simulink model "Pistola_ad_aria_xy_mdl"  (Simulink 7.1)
settings: Solver=ode45  StartTime=0.0  StopTime=10.0  RelTol=1e-6
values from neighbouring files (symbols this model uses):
  A0 = 2*cm^2    (= 0.0002)    [Pistola_ad_aria_xy.m]
  AngS = 10*gradi    (= 0.174532925199)    [Pistola_ad_aria_xy.m]
  Ap = 0.3*cm^2    (= 3e-05)    [Pistola_ad_aria_xy.m]
  b0 = 0.8*N/(10*cm/sec)    (= 8)    [Pistola_ad_aria_xy.m]
  Bp = eye(2)*bp    [Pistola_ad_aria_xy.m]
  bt = bm+b1*(r0/r1)^2+b3*(r0*r2/(r1*r3))^2+b5*(r0*r2*r4/(r1*r3*r5))^2    (= 0.0109583333333)    [Pistola_ad_aria_xy.m]
  g = 9.81*m/sec^2    (= 9.81)    [Pistola_ad_aria_xy.m]
  Imax = 10000*Amp    (= 10000)    [Pistola_ad_aria_xy.m]
  Jt = Jm+J1*(r0/r1)^2+J3*(r0*r2/(r1*r3))^2+J5*(r0*r2*r4/(r1*r3*r5))^2    (= 3.6984375e-05)    [Pistola_ad_aria_xy.m]
  K0 = 1*800*N/(5*cm)    (= 16000)    [Pistola_ad_aria_xy.m]
  K7 = 100*N/(1*mm)    (= 100000)    [Pistola_ad_aria_xy.m]
  Ke = 0.5*N*m/Amp    (= 0.5)    [Pistola_ad_aria_xy.m]
  La = 0.05*Henry    (= 0.05)    [Pistola_ad_aria_xy.m]
  m0 = 50*gr    (= 0.05)    [Pistola_ad_aria_xy.m]
  mp = 10*gr    (= 0.01)    [Pistola_ad_aria_xy.m]
  Mp = eye(2)*mp    [Pistola_ad_aria_xy.m]
  P0 = 1*bar    (= 100000)    [Pistola_ad_aria_xy.m]
  r6 = 3.5*r0    (= 0.035)    [Pistola_ad_aria_xy.m]
  Ra = 2*Ohm    (= 2)    [Pistola_ad_aria_xy.m]
  rt = r0*r2*r4/(r1*r3*r5)    (= 0.0416666666667)    [Pistola_ad_aria_xy.m]
  Tau_r = 0*N*m    (= 0)    [Pistola_ad_aria_xy.m]
  Tc = Tfin/8000    (= 0.000625)    [Pistola_ad_aria_xy.m]
  Th3_0 = 0    [Pistola_ad_aria_xy.m]
  V0 = pi*r6*A0    (= 2.19911485751e-05)    [Pistola_ad_aria_xy.m]
  Va = 30*V    (= 30)    [Pistola_ad_aria_xy.m]
  XP_0 = [0; 1.5]*m    [Pistola_ad_aria_xy.m]

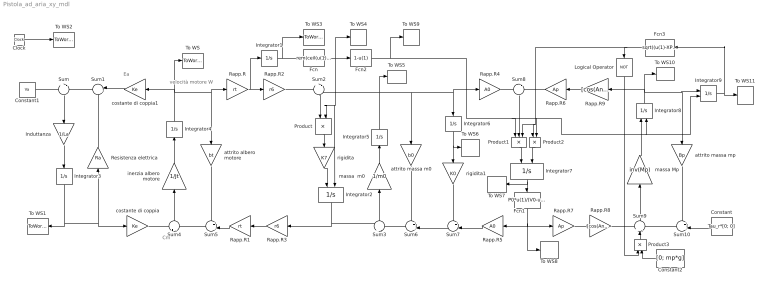
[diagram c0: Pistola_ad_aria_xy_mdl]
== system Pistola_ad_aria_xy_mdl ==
  note: Ea
  note: velocità motore W
  note: Cm
  Clock : Clock
  Constant : Constant  Orientation=left  Value=Tau_r*[0; 0]  OutDataType=sfix(16)  OutScaling=2^0
  Constant1 : Constant  Value=Va  OutDataType=sfix(16)  OutScaling=2^0
  Constant2 : Constant  Orientation=left  Value=[0; mp*g]  OutDataType=sfix(16)  OutScaling=2^0
  Fcn : Fcn  Expr=rem(ceil(u(1)/pi),2)
  Fcn1 : Fcn  Orientation=down  Expr=P0*u(1)/(V0-u(1))
  Fcn2 : Fcn  Expr=1-u(1)
  Fcn3 : Fcn  Orientation=left  Expr=sqrt((u(1)-XP_0(1))^2+(u(2)-XP_0(2))^2)<Lung_Canna
  Induttanza : Gain  Orientation=down  Gain=1/La  ParameterDataType=sfix(16)  ParameterScaling=2^0  OutDataType=sfix(16)  OutScaling=2^0
  Integrator1 : Integrator  InitialCondition=Th3_0
  Integrator2 : Integrator  Orientation=down  ExternalReset=falling
  Integrator3 : Integrator  Orientation=down  UpperSaturationLimit=Imax  LowerSaturationLimit=-Imax
  Integrator4 : Integrator  Orientation=up
  Integrator5 : Integrator  Orientation=up
  Integrator6 : Integrator  Orientation=down
  Integrator7 : Integrator  Orientation=down  ExternalReset=either
  Integrator8 : Integrator  Orientation=up  ExternalReset=rising
  Integrator9 : Integrator  ExternalReset=rising  InitialCondition=XP_0
  Logical Operator : Logic  Orientation=down  Operator=NOT  AllPortsSameDT=off  OutDataTypeMode=boolean  OutDataTypeStr=boolean
  Product : Product  Orientation=down  OutDataType=sfix(16)  OutScaling=2^0
  Product1 : Product  Orientation=down  Inputs=3  OutDataType=sfix(16)  OutScaling=2^0
  Product2 : Product  Orientation=down  OutDataType=sfix(16)  OutScaling=2^0
  Product3 : Product  Orientation=up  OutDataType=sfix(16)  OutScaling=2^0
  Rapp.R : Gain  Gain=rt  ParameterDataType=sfix(16)  ParameterScaling=2^0  OutDataType=sfix(16)  OutScaling=2^0
  Rapp.R1 : Gain  Orientation=left  Gain=rt  ParameterDataType=sfix(16)  ParameterScaling=2^0  OutDataType=sfix(16)  OutScaling=2^0
  Rapp.R2 : Gain  Gain=r6  ParameterDataType=sfix(16)  ParameterScaling=2^0  OutDataType=sfix(16)  OutScaling=2^0
  Rapp.R3 : Gain  Orientation=left  Gain=r6  ParameterDataType=sfix(16)  ParameterScaling=2^0  OutDataType=sfix(16)  OutScaling=2^0
  Rapp.R4 : Gain  Gain=A0  ParameterDataType=sfix(16)  ParameterScaling=2^0  OutDataType=sfix(16)  OutScaling=2^0
  Rapp.R5 : Gain  Orientation=left  Gain=A0  ParameterDataType=sfix(16)  ParameterScaling=2^0  OutDataType=sfix(16)  OutScaling=2^0
  Rapp.R6 : Gain  Orientation=left  Gain=Ap  ParameterDataType=sfix(16)  ParameterScaling=2^0  OutDataType=sfix(16)  OutScaling=2^0
  Rapp.R7 : Gain  Gain=Ap  ParameterDataType=sfix(16)  ParameterScaling=2^0  OutDataType=sfix(16)  OutScaling=2^0
  Rapp.R8 : Gain  Gain=[cos(AngS); sin(AngS)]  Multiplication=Matrix(K*u)  ParameterDataType=sfix(16)  ParameterScaling=2^0  OutDataType=sfix(16)  OutScaling=2^0
  Rapp.R9 : Gain  Orientation=left  Gain="[cos(AngS)  sin(AngS)]"  Multiplication=Matrix(K*u)  ParameterDataType=sfix(16)  ParameterScaling=2^0  OutDataType=sfix(16)  OutScaling=2^0
  Resistenza elettrica : Gain  Orientation=up  Gain=Ra  ParameterDataType=sfix(16)  ParameterScaling=2^0  OutDataType=sfix(16)  OutScaling=2^0
  Sum : Sum  Orientation=down  Inputs=+|-  OutDataType=sfix(16)  OutScaling=2^0
  Sum1 : Sum  Orientation=left  Inputs=|++  OutDataType=sfix(16)  OutScaling=2^0
  Sum10 : Sum  Orientation=left  Inputs=++|  OutDataType=sfix(16)  OutScaling=2^0
  Sum2 : Sum  Orientation=down  Inputs=+|-  OutDataType=sfix(16)  OutScaling=2^0
  Sum3 : Sum  Orientation=up  Inputs=+|-  OutDataType=sfix(16)  OutScaling=2^0
  Sum4 : Sum  Orientation=up  Inputs=+|-  OutDataType=sfix(16)  OutScaling=2^0
  Sum5 : Sum  Orientation=left  Inputs=++|  OutDataType=sfix(16)  OutScaling=2^0
  Sum6 : Sum  Orientation=left  Inputs=++|  OutDataType=sfix(16)  OutScaling=2^0
  Sum7 : Sum  Orientation=left  Inputs=+-|  OutDataType=sfix(16)  OutScaling=2^0
  Sum8 : Sum  Orientation=down  Inputs=-|-  OutDataType=sfix(16)  OutScaling=2^0
  Sum9 : Sum  Orientation=up  Inputs=+--  OutDataType=sfix(16)  OutScaling=2^0
  To WS : ToWorkspace  VariableName=Wm  SampleTime=Tc  SaveFormat=Array
  To WS1 : ToWorkspace  VariableName=Ia  SampleTime=Tc  SaveFormat=Array
  To WS10 : ToWorkspace  VariableName=XPdot  SampleTime=Tc  SaveFormat=Array
  To WS11 : ToWorkspace  VariableName=XP  SampleTime=Tc  SaveFormat=Array
  To WS2 : ToWorkspace  VariableName=t  SampleTime=Tc  SaveFormat=Array
  To WS3 : ToWorkspace  VariableName=Th3  SampleTime=Tc  SaveFormat=Array
  To WS4 : ToWorkspace  VariableName=Car  SampleTime=Tc  SaveFormat=Array
  To WS5 : ToWorkspace  VariableName=X0dot  SampleTime=Tc  SaveFormat=Array
  To WS6 : ToWorkspace  VariableName=X0  SampleTime=Tc  SaveFormat=Array
  To WS7 : ToWorkspace  VariableName=Vx  SampleTime=Tc  SaveFormat=Array
  To WS8 : ToWorkspace  VariableName=Px  SampleTime=Tc  SaveFormat=Array
  To WS9 : ToWorkspace  VariableName=Scar  SampleTime=Tc  SaveFormat=Array
  attrito albero motore : Gain  Orientation=down  Gain=bt  ParameterDataType=sfix(16)  ParameterScaling=2^0  OutDataType=sfix(16)  OutScaling=2^0
  attrito massa m0 : Gain  Orientation=down  Gain=b0  ParameterDataType=sfix(16)  ParameterScaling=2^0  OutDataType=sfix(16)  OutScaling=2^0
  attrito massa mp : Gain  Orientation=down  Gain=Bp  Multiplication=Matrix(K*u)  ParameterDataType=sfix(16)  ParameterScaling=2^0  OutDataType=sfix(16)  OutScaling=2^0
  costante di coppia : Gain  Gain=Ke  ParameterDataType=sfix(16)  ParameterScaling=2^0  OutDataType=sfix(16)  OutScaling=2^0
  costante di coppia1 : Gain  Orientation=left  Gain=Ke  ParameterDataType=sfix(16)  ParameterScaling=2^0  OutDataType=sfix(16)  OutScaling=2^0
  inerzia albero motore : Gain  Orientation=up  Gain=1/Jt  ParameterDataType=sfix(16)  ParameterScaling=2^0  OutDataType=sfix(16)  OutScaling=2^0
  massa  m0 : Gain  Orientation=up  Gain=1/m0  ParameterDataType=sfix(16)  ParameterScaling=2^0  OutDataType=sfix(16)  OutScaling=2^0
  massa Mp : Gain  Orientation=up  Gain=inv(Mp)  Multiplication=Matrix(K*u)  ParameterDataType=sfix(16)  ParameterScaling=2^0  OutDataType=sfix(16)  OutScaling=2^0
  rigidita : Gain  Orientation=down  Gain=K7  ParameterDataType=sfix(16)  ParameterScaling=2^0  OutDataType=sfix(16)  OutScaling=2^0
  rigidita1 : Gain  Orientation=down  Gain=K0  ParameterDataType=sfix(16)  ParameterScaling=2^0  OutDataType=sfix(16)  OutScaling=2^0
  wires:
  Clock/1 -> To WS2/1
  Sum/1 -> Induttanza/1
  Induttanza/1 -> Integrator3/1
  Sum1/1 -> Sum/2
  Resistenza elettrica/1 -> Sum1/2
  Sum4/1 -> inerzia albero motore/1
  inerzia albero motore/1 -> Integrator4/1
  Sum5/1 -> Sum4/2
  attrito albero motore/1 -> Sum5/1
  Integrator4/1 -> costante di coppia1/1, To WS/1, attrito albero motore/1, Rapp.R/1
  costante di coppia1/1 -> Sum1/1
  costante di coppia/1 -> Sum4/1
  Integrator3/1 -> Resistenza elettrica/1, costante di coppia/1, To WS1/1
  Constant1/1 -> Sum/1
  Rapp.R1/1 -> Sum5/2
  Rapp.R/1 -> Rapp.R2/1, Integrator1/1
  Rapp.R3/1 -> Rapp.R1/1
  Integrator1/1 -> To WS3/1, Fcn/1
  rigidita/1 -> Integrator2/1
  Rapp.R2/1 -> Sum2/1
  Integrator2/1 -> Rapp.R3/1, Sum3/1
  Fcn/1 -> To WS4/1, Product/2, Integrator2/2, Fcn2/1
  Sum2/1 -> Product/1
  Product/1 -> rigidita/1
  Sum3/1 -> massa  m0/1
  massa  m0/1 -> Integrator5/1
  Sum6/1 -> Sum3/2
  attrito massa m0/1 -> Sum6/1
  Integrator5/1 -> Sum2/2, To WS5/1, attrito massa m0/1, Integrator6/1, Rapp.R4/1
  Integrator6/1 -> rigidita1/1, To WS6/1
  rigidita1/1 -> Sum7/1
  Sum7/1 -> Sum6/2
  Rapp.R5/1 -> Sum7/2
  Integrator7/1 -> To WS7/1, Fcn1/1
  Rapp.R4/1 -> Sum8/1
  Rapp.R6/1 -> Sum8/2
  Sum9/1 -> massa Mp/1
  massa Mp/1 -> Integrator8/1
  attrito massa mp/1 -> Sum10/1
  Rapp.R7/1 -> Rapp.R8/1
  Integrator8/1 -> To WS10/1, attrito massa mp/1, Integrator9/1, Rapp.R9/1
  Constant/1 -> Sum10/2
  Fcn2/1 -> To WS9/1, Product1/1, Product2/2, Integrator8/2, Integrator9/2
  Fcn1/1 -> Rapp.R5/1, Rapp.R7/1, To WS8/1
  Integrator9/1 -> To WS11/1, Fcn3/1
  Product1/1 -> Integrator7/1
  Sum8/1 -> Product1/2
  Product2/1 -> Integrator7/2
  Fcn3/1 -> Product2/1, Product1/3, Logical Operator/1
  Rapp.R8/1 -> Sum9/1
  Rapp.R9/1 -> Rapp.R6/1
  Sum10/1 -> Sum9/3
  Product3/1 -> Sum9/2
  Constant2/1 -> Product3/2
  Logical Operator/1 -> Product3/1
